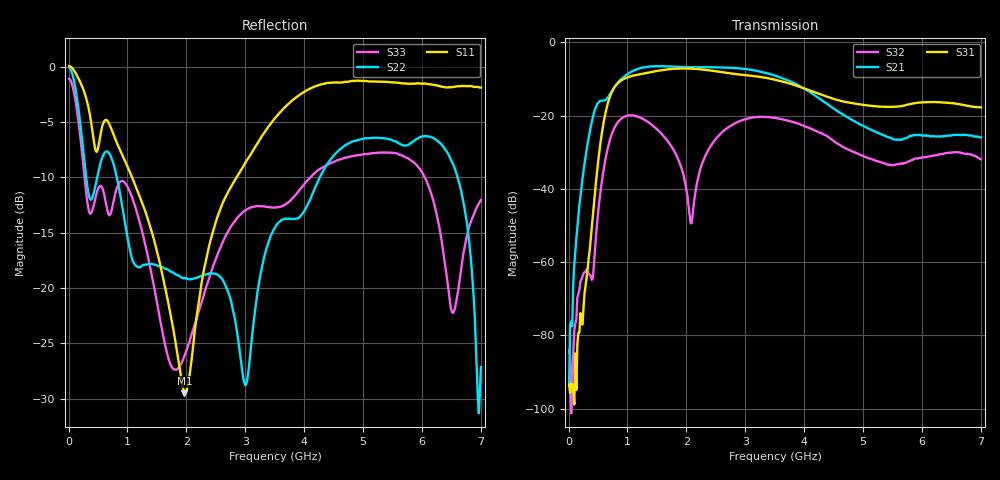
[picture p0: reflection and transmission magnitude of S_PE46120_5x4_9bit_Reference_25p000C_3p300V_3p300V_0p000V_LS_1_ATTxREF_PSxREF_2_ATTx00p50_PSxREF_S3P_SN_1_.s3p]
! Device ID: PE46120_5x4_9bit_Reference
! Device ID: PE46120_5x4_9bit_Reference
! File Path: z:\PE46120_5x4_9bit_Reference\MPAC_Yi\new_12port\25p000C\3p300\LS_1_ATTxREF_PSxREF_2_ATTx00p50_PSxREF\PE46120_5x4_9bit_Reference_25p000C_3p300V_3p300V_0p000V_LS_1_ATTxREF_PSxREF_2_ATTx00p50_PSxREF_S3P_SN_1_.s3p
! Serial: 1
! Lot:
! Temp: 25.000C
! VDD: 3.300
! VSS: 0.000
! Control_Hi: 3.300
! Control_Lo: 0.000
! Logic State: LS_1_ATTxREF_PSxREF_2_ATTx00p50_PSxREF
! Port 1: RFin
! Port 2: RFout1
! Port 3: RFout2
! ThroughPath:1-3
! IDD: -0.0005479308
! ISS: 0
! Comment:
#  Hz  S  RI  R  50
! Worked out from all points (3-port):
!   401 points, 10 MHz to 7 GHz, reference 50 ohm
!   strongest paths, dB at 10 MHz, 1.758 GHz, 3.505 GHz, 5.253 GHz, 7 GHz:
!     S31: -93.4, -7.3, -10.2, -17.5, -17.8
!     S21: -93.7, -6.7, -9.1, -24.8, -26.0
!     S32: -84.1, -28.7, -20.6, -32.5, -32.0
!   lowest |S11| = -29.5 dB at 1.967 GHz (marker M1), VSWR 1.07, Z = 52.5 + j2.3 ohm
!   |S11| at or under -10 dB: 1.079 GHz to 2.85 GHz (1.771 GHz wide, 90.2 % of centre)
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1e7  1.001 -0.1148  7.85e-05 -3.4e-05  9.48e-05 0.000116
     -1.91e-05 7.86e-06  0.9873 -0.0963  9.42e-07 9.46e-05
     -3.15e-06 -2.12e-05  4.98e-07 6.25e-05  0.8795 -0.0856
2.197e8  -0.4013 -0.7258  -0.00958 -0.0044  9.84e-06 0.000231
         -0.00965 -0.0043  -0.242 -0.4356  -0.000301 0.000438
         -6.82e-06 0.000146  -0.000299 0.000496  -0.2076 -0.3802
4.6435e8  -0.4082 -0.0743  -0.0553 0.1161  0.0113 0.00336
          -0.0557 0.1177  0.1375 0.2642  -0.00165 0.00142
          0.0115 0.00334  -0.00159 0.00145  0.1438 0.2173
9.187e8  -0.303 0.2555  0.3226 -0.0211  -0.1431 0.27
         0.3267 -0.0218  -0.0362 -0.2255  -0.0675 0.0631
         -0.1443 0.2733  -0.0682 0.0639  0.1436 -0.2684
1.9672e9  0.0252 0.0219  -0.3773 0.2489  -0.2485 -0.3553
          -0.3814 0.2523  -0.0936 0.0593  0.00103 0.0133
          -0.2521 -0.3586  0.00107 0.0135  -0.0492 -0.00123
2.806e9  -0.0796 -0.2912  0.4308 0.0913  -0.0884 0.3555
         0.436 0.0914  0.071 -0.0282  0.0125 0.0748
         -0.0886 0.3602  0.0125 0.0758  0.0666 0.1862
3.505e9  -0.4367 -0.3912  -0.0914 -0.3333  0.3014 0.0434
         -0.0925 -0.338  0.0628 0.1768  0.00925 -0.0913
         0.305 0.0433  0.00927 -0.0924  0.1657 -0.1613
4.58845e9  -0.8469 0.0498  -0.0116 0.1099  -0.0652 -0.1447
           -0.0115 0.1107  -0.3963 0.1378  0.0263 0.0293
           -0.0664 -0.1463  0.027 0.0299  -0.2441 0.2916
6.26605e9  -0.3621 0.7387  0.0386 -0.033  -0.00822 0.1499
           0.039 -0.0342  0.4482 -0.1093  -0.0283 -0.00354
           -0.00803 0.152  -0.0286 -0.00399  0.175 -0.1061
7e9  -0.1099 0.7984  -0.0294 -0.0396  0.1167 0.0503
     -0.03 -0.0401  -0.0344 0.0273  0.0248 0.00751
     0.1191 0.0504  0.024 0.00778  0.1429 0.2048
